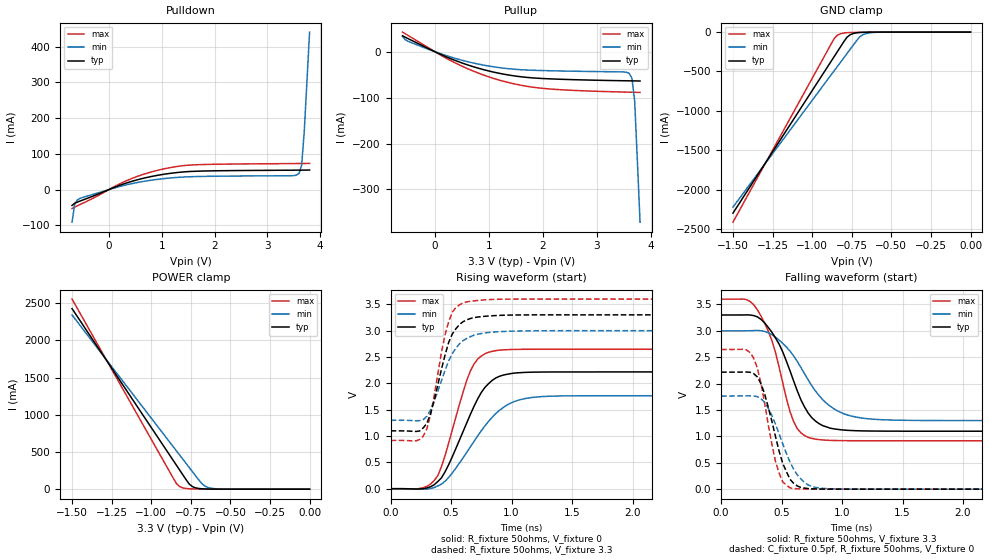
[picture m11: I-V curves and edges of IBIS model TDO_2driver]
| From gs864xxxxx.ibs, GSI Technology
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|  signals   TDO
[Model]   TDO_2driver
Model_type   3-state
Polarity   Non-Inverting
Vmeas =   1.5v
Cref  =   0pF
Rref  =   50
Vref  =   1.5v
|  variable   typ   min   max
C_comp   3.0pF   2.5pF   3.5pF
|  variable   typ   min   max
[Temperature Range]   50   0   100
|  variable   typ   min   max
[Voltage Range]   3.3   3.0   3.6
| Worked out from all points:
|   slope of the pulldown table from 0 to 0.495 V, typ, clamps not added: 19.3 ohm
|   slope of the pullup table from 0 to 0.495 V, typ, clamps not added: 20.4 ohm
|   GND clamp passes 1 mA (typ) near -0.63 V on its own axis
|   POWER clamp passes 1 mA (typ) near -0.62 V on its own axis
|   rising waveform, R_fixture 50ohms, V_fixture 0: 20-80 % time 260ps typ, 336ps min, 204ps max; typ from 0 V to 2.22 V
|   rising waveform, R_fixture 50ohms, V_fixture 3.3: 20-80 % time 152ps typ, 182ps min, 133ps max; typ from 1.1 V to 3.3 V
|   falling waveform, R_fixture 50ohms, V_fixture 3.3: 20-80 % time 244ps typ, 313ps min, 196ps max; typ from 3.3 V to 1.1 V
|   falling waveform, C_fixture 0.5pf, R_fixture 50ohms, V_fixture 0: 20-80 % time 155ps typ, 191ps min, 131ps max; typ from 2.22 V to 0 V
[Pulldown]
| voltage   I(typ)   I(min)   I(max)
-700mV    -44.39mA   -91.37mA   -53.09mA
-650mV    -38.49mA   -41.6mA    -49.27mA
-600mV    -35.14mA   -29.08mA   -45.61mA
400mV     21.52mA    15.5mA     29.04mA
900mV     39.28mA    28.18mA    53.06mA
1.45V     49.77mA    35.34mA    67.52mA
3.45V     54.18mA    38.76mA    72.68mA
3.55V     54.28mA    40.16mA    72.8mA
3.6V      54.33mA    45.16mA    72.86mA
3.65V     54.38mA    68.14mA    72.93mA
3.7V      54.44mA    164.6mA    73mA
3.8V      54.62mA    440.8mA    73.15mA
[Pullup]
| voltage (VDDQ-Vout) I(typ)   I(min)   I(max)
-600mV    34.69mA    33.37mA    42.69mA
-500mV    28.65mA    22.88mA    35.55mA
250mV     -13.12mA   -10.04mA   -16.72mA
750mV     -34.08mA   -25.63mA   -44.07mA
1.3V      -49.46mA   -36.21mA   -65.28mA
2.1V      -58.97mA   -41.37mA   -80.91mA
3.5V      -63.24mA   -44.14mA   -87.85mA
3.6V      -63.43mA   -47.18mA   -88.12mA
3.65V     -63.52mA   -58.03mA   -88.26mA
3.7V      -63.61mA   -106.8mA   -88.38mA
3.75V     -63.71mA   -236.1mA   -88.51mA
3.8V      -63.83mA   -371.2mA   -88.63mA
[GND Clamp]
| voltage   I(typ)   I(min)   I(max)
-1.5V     -2.3A      -2.224A    -2.415A
-880mV    -370.6mA   -543.1mA   -151.1mA
-860mV    -308.5mA   -489mA     -80.12mA
-840mV    -246.5mA   -434.9mA   -38.91mA
-820mV    -184.4mA   -380.9mA   -20.22mA
-780mV    -65.55mA   -272.8mA   -7.662mA
-760mV    -33.81mA   -218.9mA   -5.572mA
-700mV    -5.364mA   -62.59mA   -2.825mA
-660mV    -1.94mA    -18.77mA   -1.788mA
-560mV    -225.3uA   -949.8uA   -330.3uA
0V        -120.2pA   -376.6pA   -72.24pA
[POWER Clamp]
| voltage (VDDQ-Vout) I(typ)   I(min)   I(max)
-1.5V     2.426A     2.341A     2.554A
-860mV    382.9mA    567.6mA    145.1mA
-840mV    319.2mA    512.3mA    73.64mA
-820mV    255.5mA    457.1mA    33.99mA
-800mV    191.9mA    401.8mA    16.54mA
-760mV    68.92mA    291.3mA    5.271mA
-740mV    34.64mA    236.1mA    3.556mA
-680mV    4.879mA    73.28mA    1.644mA
-640mV    1.574mA    21.56mA    1.043mA
-540mV    157.9uA    1.034mA    211.3uA
0V        183.6pA    671.2pA    79.69pA
[Ramp]
| voltage   typ   min   max
dV/dt_r   1.33/241p   1.13/295p   1.59/197p
dV/dt_f   1.32/240p   1.13/294p   1.57/196p
R_load  =   50ohms
[Rising Waveform]
C_fixture =   0.0pf
R_fixture =   50ohms
V_fixture =   0
| Time   V(typ)   V(min)   V(max)
0s        1.439nV    5.733nV    681.5pV
270ps     -173.4uV   -8.775mV   19.66mV
390ps     135.6mV    52.68mV    245.6mV
480ps     456.6mV    213.8mV    869.6mV
660ps     1.414V     798.2mV    2.238V
720ps     1.706V     1.004V     2.461V
810ps     1.995V     1.28V      2.59V
990ps     2.184V     1.622V     2.642V
1.2ns     2.213V     1.739V     2.647V
2.97ns    2.217V     1.765V     2.647V
[Rising Waveform]
C_fixture =   0.0pf
R_fixture =   50ohms
V_fixture =   3.3
V_fixture_min =   3.0
V_fixture_max =   3.6
| Time   V(typ)   V(min)   V(max)
0s        1.098V     1.299V     916.6mV
210ps     1.087V     1.289V     909.1mV
270ps     1.155V     1.313V     999.4mV
330ps     1.425V     1.494V     1.401V
420ps     2.265V     2.048V     2.583V
480ps     2.778V     2.427V     3.171V
510ps     2.937V     2.567V     3.353V
600ps     3.172V     2.811V     3.529V
990ps     3.296V     2.99V      3.599V
2.97ns    3.3V       3V         3.6V
[Falling Waveform]
C_fixture =   0.0pf
R_fixture =   50ohms
V_fixture =   3.3
V_fixture_min =   3.0
V_fixture_max =   3.6
| Time   V(typ)   V(min)   V(max)
0s        3.3V       3V         3.6V
210ps     3.302V     3.001V     3.592V
300ps     3.265V     3.007V     3.399V
420ps     2.973V     2.927V     2.819V
510ps     2.599V     2.762V     2.013V
600ps     2.049V     2.524V     1.279V
720ps     1.442V     2.071V     981.7mV
900ps     1.157V     1.575V     924.9mV
1.17ns    1.104V     1.345V     917.2mV
2.97ns    1.098V     1.299V     916.6mV
[Falling Waveform]
C_fixture =   0.5pf
R_fixture =   50ohms
V_fixture =   0
| Time   V(typ)   V(min)   V(max)
0s        2.217V     1.765V     2.647V
210ps     2.22V      1.768V     2.638V
270ps     2.188V     1.766V     2.481V
360ps     1.805V     1.643V     1.634V
450ps     994.8mV    1.23V      523.6mV
510ps     487.4mV    857.3mV    136.6mV
570ps     185.8mV    515mV      24.2mV
690ps     21.09mV    126.8mV    3.007mV
840ps     2.501mV    15.58mV    437.8uV
2.97ns    169.4nV    486.1nV    64.99nV
